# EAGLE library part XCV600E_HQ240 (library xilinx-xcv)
xcv600e_hq240 edit this description Auto generated by make-symbol-device-package-bsdl.ulp Rev. 26 Source: xcv600e_hq240.bsd
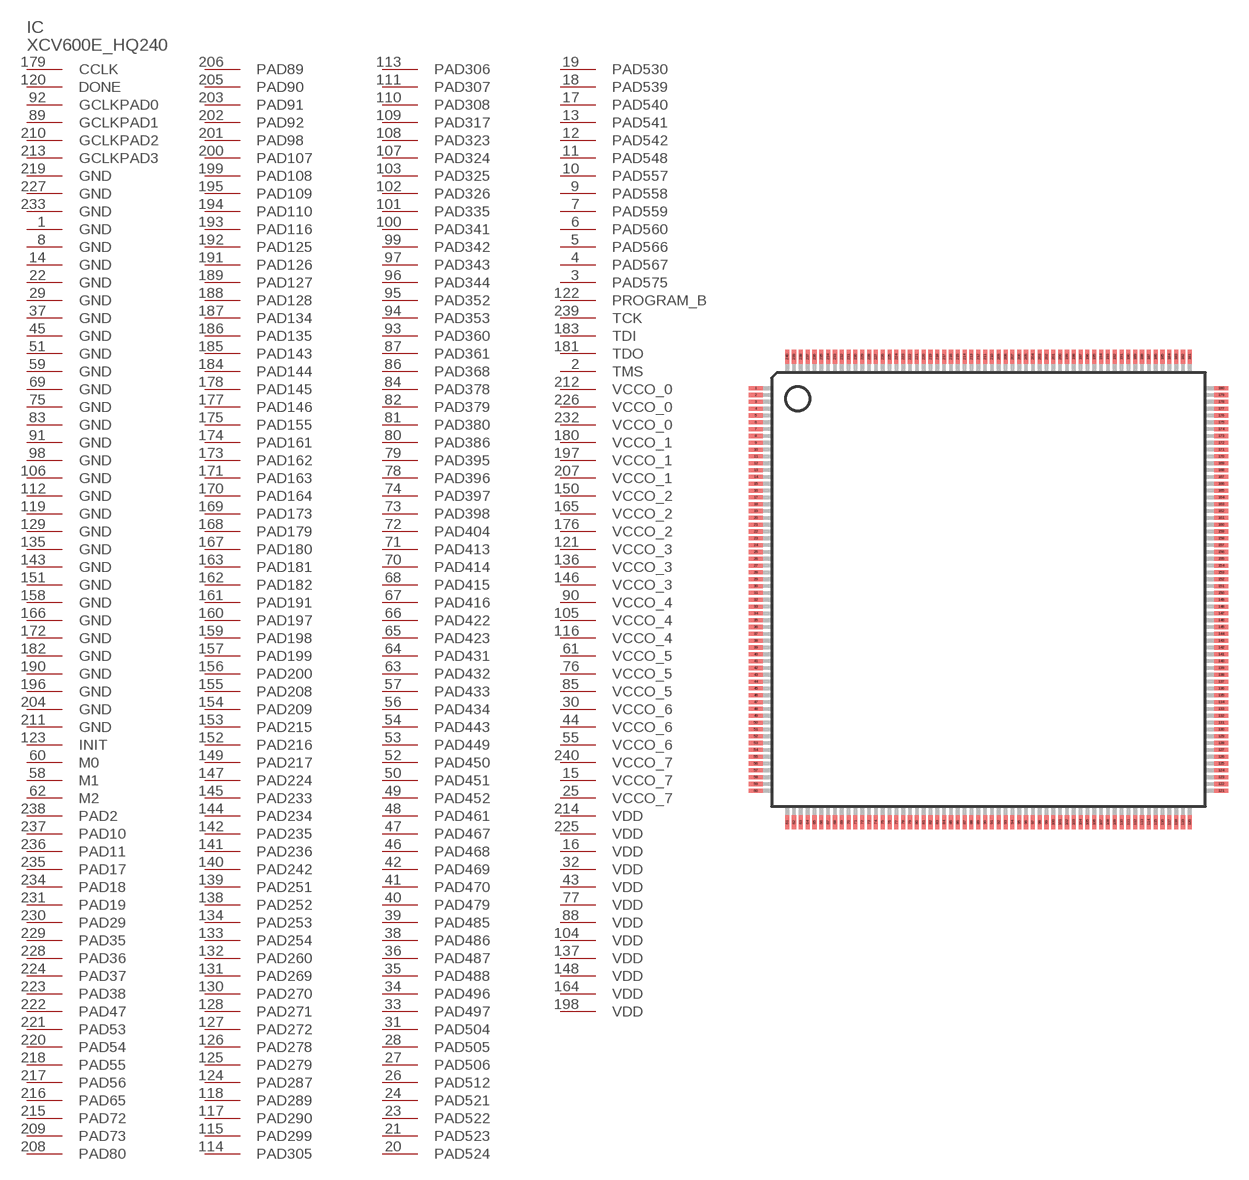
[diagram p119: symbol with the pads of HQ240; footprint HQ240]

Designator prefix IC

## XCV600E_HQ240 (OC_FARNELL: unknown; OC_NEWARK: unknown)  [HQ240]
1  GND  pwr
2  TMS  in
3  PAD575
4  PAD567
5  PAD566
6  PAD560
7  PAD559
8  GND  pwr
9  PAD558
10  PAD557
11  PAD548
12  PAD542
13  PAD541
14  GND  pwr
15  VCCO_7  pwr
16  VDD  pwr
17  PAD540
18  PAD539
19  PAD530
20  PAD524
21  PAD523
22  GND  pwr
23  PAD522
24  PAD521
25  VCCO_7  pwr
26  PAD512
27  PAD506
28  PAD505
29  GND  pwr
30  VCCO_6  pwr
31  PAD504
32  VDD  pwr
33  PAD497
34  PAD496
35  PAD488
36  PAD487
37  GND  pwr
38  PAD486
39  PAD485
40  PAD479
41  PAD470
42  PAD469
43  VDD  pwr
44  VCCO_6  pwr
45  GND  pwr
46  PAD468
47  PAD467
48  PAD461
49  PAD452
50  PAD451
51  GND  pwr
52  PAD450
53  PAD449
54  PAD443
55  VCCO_6  pwr
56  PAD434
57  PAD433
58  M1  in
59  GND  pwr
60  M0  in
61  VCCO_5  pwr
62  M2  in
63  PAD432
64  PAD431
65  PAD423
66  PAD422
67  PAD416
68  PAD415
69  GND  pwr
70  PAD414
71  PAD413
72  PAD404
73  PAD398
74  PAD397
75  GND  pwr
76  VCCO_5  pwr
77  VDD  pwr
78  PAD396
79  PAD395
80  PAD386
81  PAD380
82  PAD379
83  GND  pwr
84  PAD378
85  VCCO_5  pwr
86  PAD368
87  PAD361
88  VDD  pwr
89  GCLKPAD1  in
90  VCCO_4  pwr
91  GND  pwr
92  GCLKPAD0  in
93  PAD360
94  PAD353
95  PAD352
96  PAD344
97  PAD343
98  GND  pwr
99  PAD342
100  PAD341
101  PAD335
102  PAD326
103  PAD325
104  VDD  pwr
105  VCCO_4  pwr
106  GND  pwr
107  PAD324
108  PAD323
109  PAD317
110  PAD308
111  PAD307
112  GND  pwr
113  PAD306
114  PAD305
115  PAD299
116  VCCO_4  pwr
117  PAD290
118  PAD289
119  GND  pwr
120  DONE
121  VCCO_3  pwr
122  PROGRAM_B  in
123  INIT
124  PAD287
125  PAD279
126  PAD278
127  PAD272
128  PAD271
129  GND  pwr
130  PAD270
131  PAD269
132  PAD260
133  PAD254
134  PAD253
135  GND  pwr
136  VCCO_3  pwr
137  VDD  pwr
138  PAD252
139  PAD251
140  PAD242
141  PAD236
142  PAD235
143  GND  pwr
144  PAD234
145  PAD233
146  VCCO_3  pwr
147  PAD224
148  VDD  pwr
149  PAD217
150  VCCO_2  pwr
151  GND  pwr
152  PAD216
153  PAD215
154  PAD209
155  PAD208
156  PAD200
157  PAD199
158  GND  pwr
159  PAD198
160  PAD197
161  PAD191
162  PAD182
163  PAD181
164  VDD  pwr
165  VCCO_2  pwr
166  GND  pwr
167  PAD180
168  PAD179
169  PAD173
170  PAD164
171  PAD163
172  GND  pwr
173  PAD162
174  PAD161
175  PAD155
176  VCCO_2  pwr
177  PAD146
178  PAD145
179  CCLK
180  VCCO_1  pwr
181  TDO  out
182  GND  pwr
183  TDI  in
184  PAD144
185  PAD143
186  PAD135
187  PAD134
188  PAD128
189  PAD127
190  GND  pwr
191  PAD126
192  PAD125
193  PAD116
194  PAD110
195  PAD109
196  GND  pwr
197  VCCO_1  pwr
198  VDD  pwr
199  PAD108
200  PAD107
201  PAD98
202  PAD92
203  PAD91
204  GND  pwr
205  PAD90
206  PAD89
207  VCCO_1  pwr
208  PAD80
209  PAD73
210  GCLKPAD2  in
211  GND  pwr
212  VCCO_0  pwr
213  GCLKPAD3  in
214  VDD  pwr
215  PAD72
216  PAD65
217  PAD56
218  PAD55
219  GND  pwr
220  PAD54
221  PAD53
222  PAD47
223  PAD38
224  PAD37
225  VDD  pwr
226  VCCO_0  pwr
227  GND  pwr
228  PAD36
229  PAD35
230  PAD29
231  PAD19
232  VCCO_0  pwr
233  GND  pwr
234  PAD18
235  PAD17
236  PAD11
237  PAD10
238  PAD2
239  TCK  in
240  VCCO_7  pwr

## Footprint HQ240 (pad centres in mm)
HQ240 Auto generated by make-symbol-device-package-bsdl.ulp Rev. 26
smd 1 x 0.3: 1 -17.05,14.75; 2 -17.05,14.25; 3 -17.05,13.75; 4 -17.05,13.25; 5 -17.05,12.75; 6 -17.05,12.25; 7 -17.05,11.75; 8 -17.05,11.25; 9 -17.05,10.75; 10 -17.05,10.25; 11 -17.05,9.75; 12 -17.05,9.25; 13 -17.05,8.75; 14 -17.05,8.25; 15 -17.05,7.75; 16 -17.05,7.25; 17 -17.05,6.75; 18 -17.05,6.25; 19 -17.05,5.75; 20 -17.05,5.25; 21 -17.05,4.75; 22 -17.05,4.25; 23 -17.05,3.75; 24 -17.05,3.25; 25 -17.05,2.75; 26 -17.05,2.25; 27 -17.05,1.75; 28 -17.05,1.25; 29 -17.05,0.75; 30 -17.05,0.25; 31 -17.05,-0.25; 32 -17.05,-0.75; 33 -17.05,-1.25; 34 -17.05,-1.75; 35 -17.05,-2.25; 36 -17.05,-2.75; 37 -17.05,-3.25; 38 -17.05,-3.75; 39 -17.05,-4.25; 40 -17.05,-4.75; 41 -17.05,-5.25; 42 -17.05,-5.75; 43 -17.05,-6.25; 44 -17.05,-6.75; 45 -17.05,-7.25; 46 -17.05,-7.75; 47 -17.05,-8.25; 48 -17.05,-8.75; 49 -17.05,-9.25; 50 -17.05,-9.75; 51 -17.05,-10.25; 52 -17.05,-10.75; 53 -17.05,-11.25; 54 -17.05,-11.75; 55 -17.05,-12.25; 56 -17.05,-12.75; 57 -17.05,-13.25; 58 -17.05,-13.75; 59 -17.05,-14.25; 60 -17.05,-14.75; 121 17.05,-14.75; 122 17.05,-14.25; 123 17.05,-13.75; 124 17.05,-13.25; 125 17.05,-12.75; 126 17.05,-12.25; 127 17.05,-11.75; 128 17.05,-11.25; 129 17.05,-10.75; 130 17.05,-10.25; 131 17.05,-9.75; 132 17.05,-9.25; 133 17.05,-8.75; 134 17.05,-8.25; 135 17.05,-7.75; 136 17.05,-7.25; 137 17.05,-6.75; 138 17.05,-6.25; 139 17.05,-5.75; 140 17.05,-5.25; 141 17.05,-4.75; 142 17.05,-4.25; 143 17.05,-3.75; 144 17.05,-3.25; 145 17.05,-2.75; 146 17.05,-2.25; 147 17.05,-1.75; 148 17.05,-1.25; 149 17.05,-0.75; 150 17.05,-0.25; 151 17.05,0.25; 152 17.05,0.75; 153 17.05,1.25; 154 17.05,1.75; 155 17.05,2.25; 156 17.05,2.75; 157 17.05,3.25; 158 17.05,3.75; 159 17.05,4.25; 160 17.05,4.75; 161 17.05,5.25; 162 17.05,5.75; 163 17.05,6.25; 164 17.05,6.75; 165 17.05,7.25; 166 17.05,7.75; 167 17.05,8.25; 168 17.05,8.75; 169 17.05,9.25; 170 17.05,9.75; 171 17.05,10.25; 172 17.05,10.75; 173 17.05,11.25; 174 17.05,11.75; 175 17.05,12.25; 176 17.05,12.75; 177 17.05,13.25; 178 17.05,13.75; 179 17.05,14.25; 180 17.05,14.75
smd 0.3 x 1: 61 -14.75,-17.05; 62 -14.25,-17.05; 63 -13.75,-17.05; 64 -13.25,-17.05; 65 -12.75,-17.05; 66 -12.25,-17.05; 67 -11.75,-17.05; 68 -11.25,-17.05; 69 -10.75,-17.05; 70 -10.25,-17.05; 71 -9.75,-17.05; 72 -9.25,-17.05; 73 -8.75,-17.05; 74 -8.25,-17.05; 75 -7.75,-17.05; 76 -7.25,-17.05; 77 -6.75,-17.05; 78 -6.25,-17.05; 79 -5.75,-17.05; 80 -5.25,-17.05; 81 -4.75,-17.05; 82 -4.25,-17.05; 83 -3.75,-17.05; 84 -3.25,-17.05; 85 -2.75,-17.05; 86 -2.25,-17.05; 87 -1.75,-17.05; 88 -1.25,-17.05; 89 -0.75,-17.05; 90 -0.25,-17.05; 91 0.25,-17.05; 92 0.75,-17.05; 93 1.25,-17.05; 94 1.75,-17.05; 95 2.25,-17.05; 96 2.75,-17.05; 97 3.25,-17.05; 98 3.75,-17.05; 99 4.25,-17.05; 100 4.75,-17.05; 101 5.25,-17.05; 102 5.75,-17.05; 103 6.25,-17.05; 104 6.75,-17.05; 105 7.25,-17.05; 106 7.75,-17.05; 107 8.25,-17.05; 108 8.75,-17.05; 109 9.25,-17.05; 110 9.75,-17.05; 111 10.25,-17.05; 112 10.75,-17.05; 113 11.25,-17.05; 114 11.75,-17.05; 115 12.25,-17.05; 116 12.75,-17.05; 117 13.25,-17.05; 118 13.75,-17.05; 119 14.25,-17.05; 120 14.75,-17.05; 181 14.75,17.05; 182 14.25,17.05; 183 13.75,17.05; 184 13.25,17.05; 185 12.75,17.05; 186 12.25,17.05; 187 11.75,17.05; 188 11.25,17.05; 189 10.75,17.05; 190 10.25,17.05; 191 9.75,17.05; 192 9.25,17.05; 193 8.75,17.05; 194 8.25,17.05; 195 7.75,17.05; 196 7.25,17.05; 197 6.75,17.05; 198 6.25,17.05; 199 5.75,17.05; 200 5.25,17.05; 201 4.75,17.05; 202 4.25,17.05; 203 3.75,17.05; 204 3.25,17.05; 205 2.75,17.05; 206 2.25,17.05; 207 1.75,17.05; 208 1.25,17.05; 209 0.75,17.05; 210 0.25,17.05; 211 -0.25,17.05; 212 -0.75,17.05; 213 -1.25,17.05; 214 -1.75,17.05; 215 -2.25,17.05; 216 -2.75,17.05; 217 -3.25,17.05; 218 -3.75,17.05; 219 -4.25,17.05; 220 -4.75,17.05; 221 -5.25,17.05; 222 -5.75,17.05; 223 -6.25,17.05; 224 -6.75,17.05; 225 -7.25,17.05; 226 -7.75,17.05; 227 -8.25,17.05; 228 -8.75,17.05; 229 -9.25,17.05; 230 -9.75,17.05; 231 -10.25,17.05; 232 -10.75,17.05; 233 -11.25,17.05; 234 -11.75,17.05; 235 -12.25,17.05; 236 -12.75,17.05; 237 -13.25,17.05; 238 -13.75,17.05; 239 -14.25,17.05; 240 -14.75,17.05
